TYPE E_AnalysisIDs :
(
	(* analysis chain *)
	eID_Source := 1,
	eID_IntegratedRMS,
	eID_IntegratedRMS_Sink,
	eID_EmpiricalMean,
	eID_EmpiricalMean_Sink,
	eID_EmpiricalStd,
	eID_EmpiricalStd_Sink,
	eID_Classify,
	eID_Classify_Sink
) UDINT;
END_TYPE
